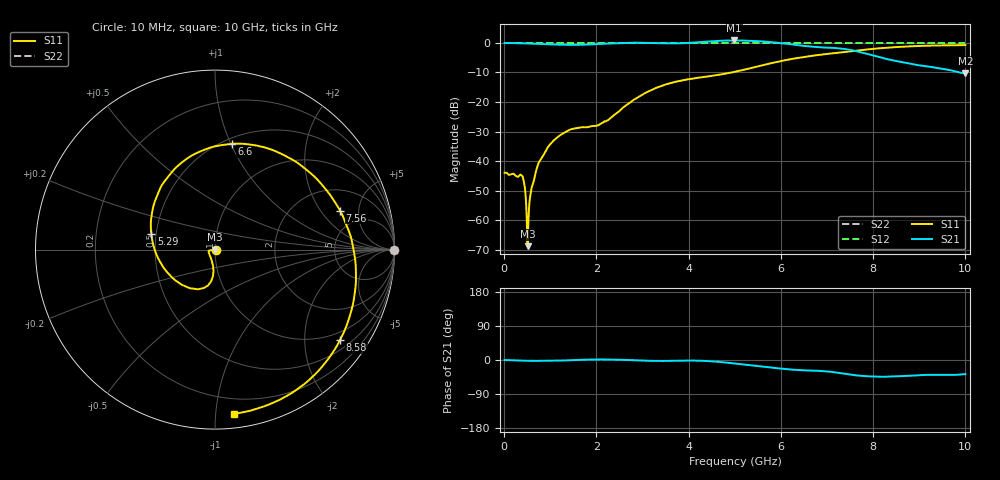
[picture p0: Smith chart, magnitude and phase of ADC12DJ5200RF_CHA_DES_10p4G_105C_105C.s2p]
! Texas Instruments, Inc.
! ADC12DJ5200RF - CH A S-Parameters (DES Mode, Fs = 10.4 GSPS, 105 degC case, 105 degC juntion)
! Port 1 represents the 100-ohm differenal input, Port 2 the digital output
! freq  dbS11  angS11  dbS21 angS21 dbS12 angS12 dbS22 angS22
# HZ S DB R 100
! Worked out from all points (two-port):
!   1000 points, 10 MHz to 10 GHz, reference 100 ohm
!   highest |S21| = 0.86 dB at 4.99 GHz (marker M1); lowest = -10.3 dB at 10 GHz (marker M2)
!   |S21| within 3 dB of the highest: start of sweep to 7.418 GHz
!   lowest |S11| = -68.9 dB at 510 MHz (marker M3), VSWR 1.00, Z = 100 - j0.0713 ohm
!   |S11| at or under -10 dB: start of sweep to 4.932 GHz
!   |S22| runs from 0.0 to 0.0 dB; largest |S21 - S12| = 0.78
!   S11 on the Smith chart (normalised r, x): 10 MHz: 1.01, -0.00; 5.29 GHz: 0.47, +0.10; 6.6 GHz: 0.55, +1.01; 7.56 GHz: 3.35, +3.13; 8.58 GHz: 0.75, -2.91; 10 GHz: 0.09, -1.12
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1e7  -43.98 -7.6  0.00 -0.0  0.00 0.0  0.00 0.0
3.8e8  -44.92 -10.5  -0.09 -1.7  0.00 0.0  0.00 0.0
4.3e8  -47.24 -0.5  -0.12 -1.9  0.00 0.0  0.00 0.0
4.7e8  -52.81 6.8  -0.14 -2.0  0.00 0.0  0.00 0.0
5.1e8  -68.87 -81.6  -0.16 -2.1  0.00 0.0  0.00 0.0
7.1e8  -42.37 -157.4  -0.31 -2.3  0.00 0.0  0.00 0.0
9.4e8  -35.52 -169.1  -0.43 -2.2  0.00 0.0  0.00 0.0
1.26e9  -30.80 -171.7  -0.60 -1.4  0.00 0.0  0.00 0.0
1.68e9  -28.56 -163.4  -0.61 0.5  0.00 0.0  0.00 0.0
2.24e9  -26.25 -119.8  -0.20 1.1  0.00 0.0  0.00 0.0
3.34e9  -14.98 -96.9  -0.04 -2.5  0.00 0.0  0.00 0.0
4.23e9  -11.74 -125.4  0.27 -1.8  0.00 0.0  0.00 0.0
4.99e9  -9.80 -173.0  0.86 -9.0  0.00 0.0  0.00 0.0
5.01e9  -9.74 -174.4  0.86 -9.3  0.00 0.0  0.00 0.0
5.29e9  -8.74 165.9  0.75 -12.8  0.00 0.0  0.00 0.0
5.9e9  -6.49 126.2  0.12 -21.4  0.00 0.0  0.00 0.0
6.6e9  -4.49 81.1  -1.12 -27.7  0.00 0.0  0.00 0.0
6.67e9  -4.33 76.5  -1.25 -28.1  0.00 0.0  0.00 0.0
7.56e9  -2.73 17.4  -2.51 -39.4  0.00 0.0  0.00 0.0
8.34e9  -1.56 -25.8  -5.59 -43.8  0.00 0.0  0.00 0.0
8.58e9  -1.31 -35.9  -6.34 -42.5  0.00 0.0  0.00 0.0
1e10  -0.71 -83.2  -10.34 -37.2  0.00 0.0  0.00 0.0
